(* Logix 5000 AddOnInstructionDefinition export AMCI_SMD23E2_Program_Assembed_Move; software revision 20.03 *)

ADD_ON_INSTRUCTION AMCI_SMD23E2_Program_Assembed_Move   (* revision 1.0, vendor AMCI *)
VAR_INPUT
   SMD23E2_Status_Word_0 : INT; {required}
        .8   // set when SMD23E2 is in Assembled Move mode
        .9   // set when the SMD23E2 is ready to receive an assembled move segment
   Number_of_Segments : DINT; {required}
   Segment_1_Distance : DINT; {required}
   Segment_1_Programmed_Speed : DINT; {required}
   Segment_1_Acceleration : INT; {required}
   Segment_1_Deceleration : INT; {required}
   Segment_2_Distance : DINT; {required}
   Segment_2_Programmed_Speed : DINT; {required}
   Segment_2_Acceleration : INT; {required}
   Segment_2_Deceleration : INT; {required}
   Segment_3_Distance : DINT; {required}
   Segment_3_Programmed_Speed : DINT; {required}
   Segment_3_Acceleration : INT; {required}
   Segment_3_Deceleration : INT; {required}
   Segment_4_Distance : DINT; {required}
   Segment_4_Programmed_Speed : DINT; {required}
   Segment_4_Acceleration : INT; {required}
   Segment_4_Deceleration : INT; {required}
   Segment_5_Distance : DINT; {required}
   Segment_5_Programmed_Speed : DINT; {required}
   Segment_5_Acceleration : INT; {required}
   Segment_5_Deceleration : INT; {required}
   Segment_6_Distance : DINT; {required}
   Segment_6_Programmed_Speed : DINT; {required}
   Segment_6_Acceleration : INT; {required}
   Segment_6_Deceleration : INT; {required}
   Segment_7_Distance : DINT; {required}
   Segment_7_Programmed_Speed : DINT; {required}
   Segment_7_Acceleration : INT; {required}
   Segment_7_Deceleration : INT; {required}
   Segment_8_Distance : DINT; {required}
   Segment_8_Programmed_Speed : DINT; {required}
   Segment_8_Acceleration : INT; {required}
   Segment_8_Deceleration : INT; {required}
   Segment_9_Distance : DINT; {required}
   Segment_9_Programmed_Speed : DINT; {required}
   Segment_9_Acceleration : INT; {required}
   Segment_9_Deceleration : INT; {required}
   Segment_10_Distance : DINT; {required}
   Segment_10_Programmed_Speed : DINT; {required}
   Segment_10_Acceleration : INT; {required}
   Segment_10_Deceleration : INT; {required}
   Segment_11_Distance : DINT; {required}
   Segment_11_Programmed_Speed : DINT; {required}
   Segment_11_Acceleration : INT; {required}
   Segment_11_Deceleration : INT; {required}
   Segment_12_Distance : DINT; {required}
   Segment_12_Programmed_Speed : DINT; {required}
   Segment_12_Acceleration : INT; {required}
   Segment_12_Deceleration : INT; {required}
   Segment_13_Distance : DINT; {required}
   Segment_13_Programmed_Speed : DINT; {required}
   Segment_13_Acceleration : INT; {required}
   Segment_13_Deceleration : INT; {required}
   Segment_14_Distance : DINT; {required}
   Segment_14_Programmed_Speed : DINT; {required}
   Segment_14_Acceleration : INT; {required}
   Segment_14_Deceleration : INT; {required}
   Segment_15_Distance : DINT; {required}
   Segment_15_Programmed_Speed : DINT; {required}
   Segment_15_Acceleration : INT; {required}
   Segment_15_Deceleration : INT; {required}
   Segment_16_Distance : DINT; {required}
   Segment_16_Programmed_Speed : DINT; {required}
   Segment_16_Acceleration : INT; {required}
   Segment_16_Deceleration : INT; {required}
END_VAR
VAR_IN_OUT
   AMCI_SMD23E2_output_data : _000A:SMD23E2_788832CB:O:0; {required}
END_VAR
VAR_OUTPUT
   Assembled_Move_Programmed : BOOL; {access Read Only, visible}
END_VAR
VAR
   command_data_block : INT[10];
        [0]   // Command Bits MSW
        [1]   // Command Bits LSW
        [2]   // Upper Target Position
        [3]   // Lower Target Position
        [4]   // Upper Programmed Speed
        [5]   // Lower Programmed Speed
   Assembled_Move_setup : INT[10] := ([0] := 2048, [1] := -32768); {access None}
   Assembled_Move_counter : COUNTER := (PRE := 5); {access None}
        .ACC   // Controls which segment is sent to the SMD23E2
   comment_coil : BOOL; {access None}
END_VAR

ROUTINE Logic   (* ladder *)
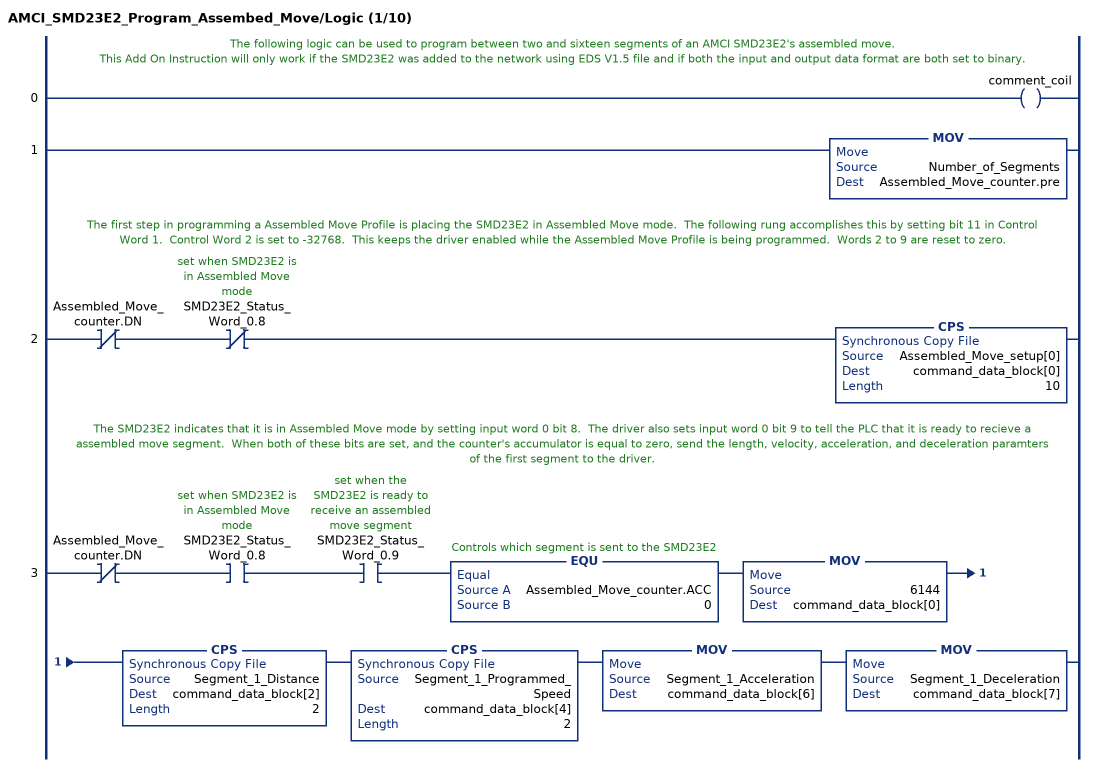
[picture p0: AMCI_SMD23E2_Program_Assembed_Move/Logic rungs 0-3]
   // The following logic can be used to program between two and sixteen segments of an AMCI SMD23E2's assembled move.
   // This Add On Instruction will only work if the SMD23E2 was added to the network using EDS V1.5 file and if both the input and output data format are both set to binary.
   0: OTE(comment_coil);
   1: MOV(Number_of_Segments,Assembled_Move_counter.pre);
   // The first step in programming a Assembled Move Profile is placing the SMD23E2 in Assembled Move mode.  The following rung accomplishes this by setting bit 11 in Control Word 1.  Control Word 2 is set to -32768.  This keeps the driver enabled while the Assembled Move Profile is being programmed.  Words 2 to 9 are reset to zero.
   2: XIO(Assembled_Move_counter.DN)XIO(SMD23E2_Status_Word_0.8)CPS(Assembled_Move_setup[0],command_data_block[0],10);
   // The SMD23E2 indicates that it is in Assembled Move mode by setting input word 0 bit 8.  The driver also sets input word 0 bit 9 to tell the PLC that it is ready to recieve a assembled move segment.  When both of these bits are set, and the counter's accumulator is equal to zero, send the length, velocity, acceleration, and deceleration paramters of the first segment to the driver.
   3: XIO(Assembled_Move_counter.DN)XIC(SMD23E2_Status_Word_0.8)XIC(SMD23E2_Status_Word_0.9)EQU(Assembled_Move_counter.ACC,0)MOV(6144,command_data_block[0])CPS(Segment_1_Distance,command_data_block[2],2)CPS(Segment_1_Programmed_Speed,command_data_block[4],2)MOV(Segment_1_Acceleration,command_data_block[6])MOV(Segment_1_Deceleration,command_data_block[7]);
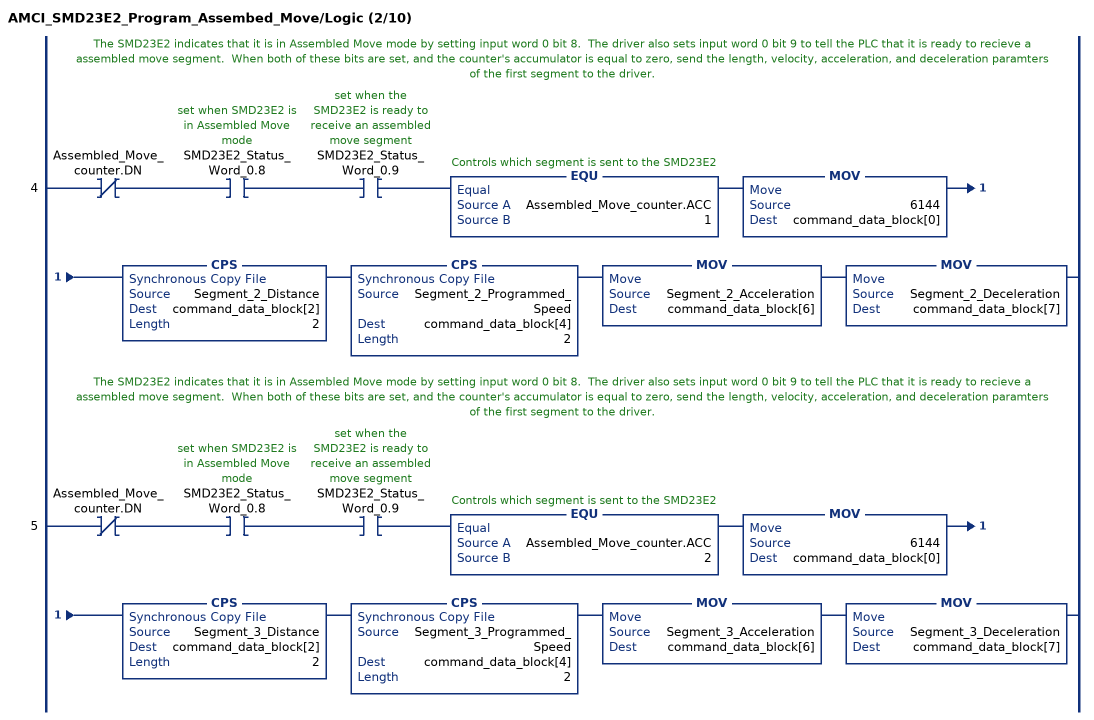
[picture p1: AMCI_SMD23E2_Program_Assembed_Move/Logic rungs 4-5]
   // The SMD23E2 indicates that it is in Assembled Move mode by setting input word 0 bit 8.  The driver also sets input word 0 bit 9 to tell the PLC that it is ready to recieve a assembled move segment.  When both of these bits are set, and the counter's accumulator is equal to zero, send the length, velocity, acceleration, and deceleration paramters of the first segment to the driver.
   4: XIO(Assembled_Move_counter.DN)XIC(SMD23E2_Status_Word_0.8)XIC(SMD23E2_Status_Word_0.9)EQU(Assembled_Move_counter.ACC,1)MOV(6144,command_data_block[0])CPS(Segment_2_Distance,command_data_block[2],2)CPS(Segment_2_Programmed_Speed,command_data_block[4],2)MOV(Segment_2_Acceleration,command_data_block[6])MOV(Segment_2_Deceleration,command_data_block[7]);
   // The SMD23E2 indicates that it is in Assembled Move mode by setting input word 0 bit 8.  The driver also sets input word 0 bit 9 to tell the PLC that it is ready to recieve a assembled move segment.  When both of these bits are set, and the counter's accumulator is equal to zero, send the length, velocity, acceleration, and deceleration paramters of the first segment to the driver.
   5: XIO(Assembled_Move_counter.DN)XIC(SMD23E2_Status_Word_0.8)XIC(SMD23E2_Status_Word_0.9)EQU(Assembled_Move_counter.ACC,2)MOV(6144,command_data_block[0])CPS(Segment_3_Distance,command_data_block[2],2)CPS(Segment_3_Programmed_Speed,command_data_block[4],2)MOV(Segment_3_Acceleration,command_data_block[6])MOV(Segment_3_Deceleration,command_data_block[7]);
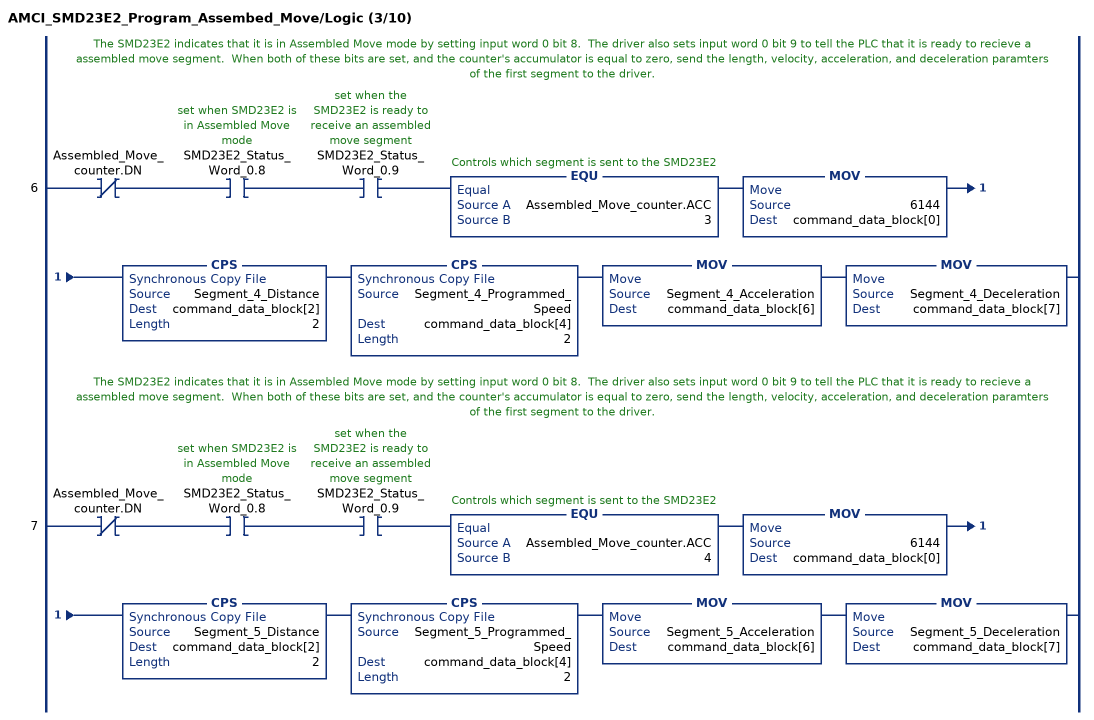
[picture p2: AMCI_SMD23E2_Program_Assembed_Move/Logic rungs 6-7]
   // The SMD23E2 indicates that it is in Assembled Move mode by setting input word 0 bit 8.  The driver also sets input word 0 bit 9 to tell the PLC that it is ready to recieve a assembled move segment.  When both of these bits are set, and the counter's accumulator is equal to zero, send the length, velocity, acceleration, and deceleration paramters of the first segment to the driver.
   6: XIO(Assembled_Move_counter.DN)XIC(SMD23E2_Status_Word_0.8)XIC(SMD23E2_Status_Word_0.9)EQU(Assembled_Move_counter.ACC,3)MOV(6144,command_data_block[0])CPS(Segment_4_Distance,command_data_block[2],2)CPS(Segment_4_Programmed_Speed,command_data_block[4],2)MOV(Segment_4_Acceleration,command_data_block[6])MOV(Segment_4_Deceleration,command_data_block[7]);
   // The SMD23E2 indicates that it is in Assembled Move mode by setting input word 0 bit 8.  The driver also sets input word 0 bit 9 to tell the PLC that it is ready to recieve a assembled move segment.  When both of these bits are set, and the counter's accumulator is equal to zero, send the length, velocity, acceleration, and deceleration paramters of the first segment to the driver.
   7: XIO(Assembled_Move_counter.DN)XIC(SMD23E2_Status_Word_0.8)XIC(SMD23E2_Status_Word_0.9)EQU(Assembled_Move_counter.ACC,4)MOV(6144,command_data_block[0])CPS(Segment_5_Distance,command_data_block[2],2)CPS(Segment_5_Programmed_Speed,command_data_block[4],2)MOV(Segment_5_Acceleration,command_data_block[6])MOV(Segment_5_Deceleration,command_data_block[7]);
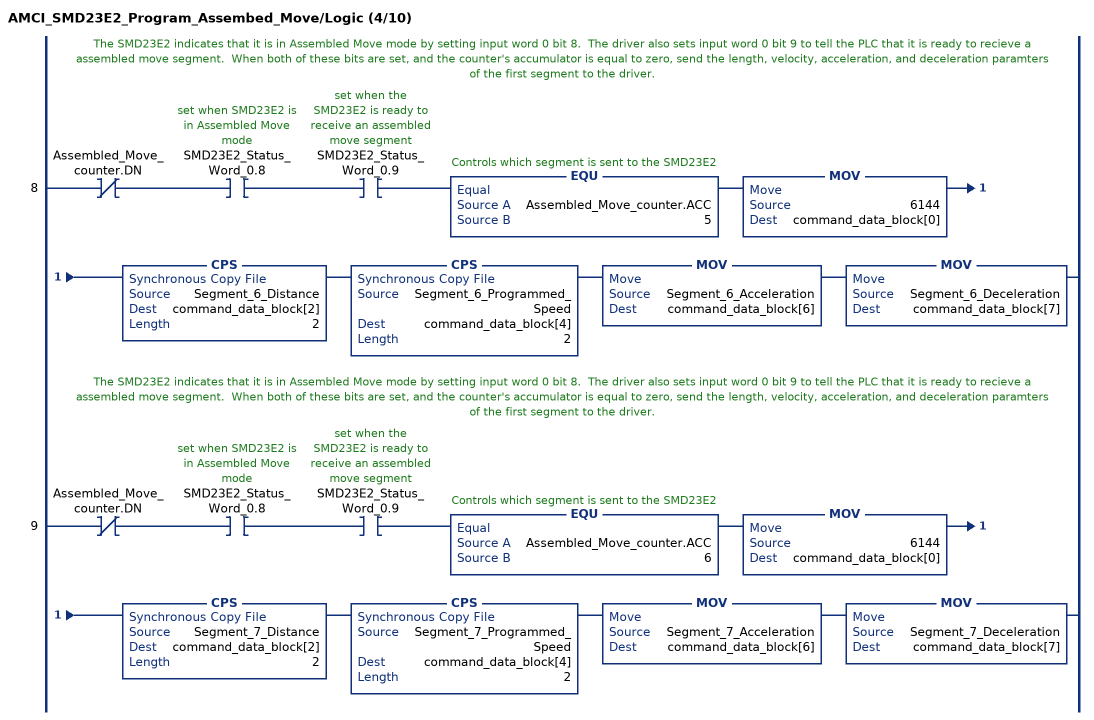
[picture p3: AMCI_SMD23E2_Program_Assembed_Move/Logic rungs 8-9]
   // The SMD23E2 indicates that it is in Assembled Move mode by setting input word 0 bit 8.  The driver also sets input word 0 bit 9 to tell the PLC that it is ready to recieve a assembled move segment.  When both of these bits are set, and the counter's accumulator is equal to zero, send the length, velocity, acceleration, and deceleration paramters of the first segment to the driver.
   8: XIO(Assembled_Move_counter.DN)XIC(SMD23E2_Status_Word_0.8)XIC(SMD23E2_Status_Word_0.9)EQU(Assembled_Move_counter.ACC,5)MOV(6144,command_data_block[0])CPS(Segment_6_Distance,command_data_block[2],2)CPS(Segment_6_Programmed_Speed,command_data_block[4],2)MOV(Segment_6_Acceleration,command_data_block[6])MOV(Segment_6_Deceleration,command_data_block[7]);
   // The SMD23E2 indicates that it is in Assembled Move mode by setting input word 0 bit 8.  The driver also sets input word 0 bit 9 to tell the PLC that it is ready to recieve a assembled move segment.  When both of these bits are set, and the counter's accumulator is equal to zero, send the length, velocity, acceleration, and deceleration paramters of the first segment to the driver.
   9: XIO(Assembled_Move_counter.DN)XIC(SMD23E2_Status_Word_0.8)XIC(SMD23E2_Status_Word_0.9)EQU(Assembled_Move_counter.ACC,6)MOV(6144,command_data_block[0])CPS(Segment_7_Distance,command_data_block[2],2)CPS(Segment_7_Programmed_Speed,command_data_block[4],2)MOV(Segment_7_Acceleration,command_data_block[6])MOV(Segment_7_Deceleration,command_data_block[7]);
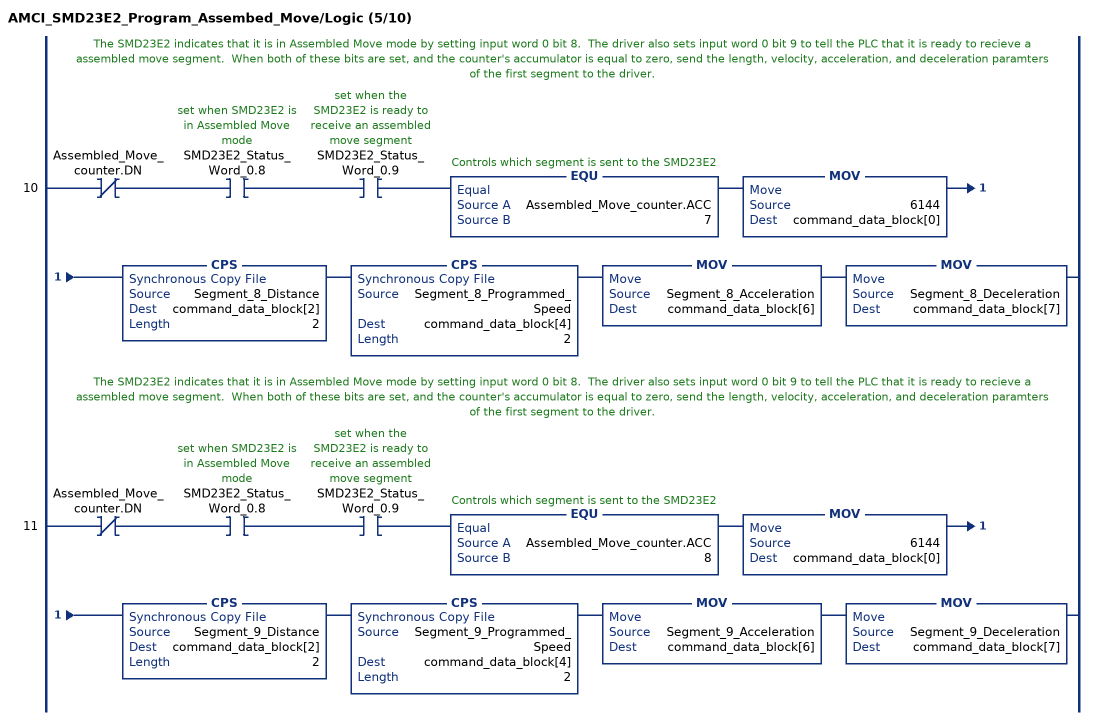
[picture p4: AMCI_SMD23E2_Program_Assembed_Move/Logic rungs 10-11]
   // The SMD23E2 indicates that it is in Assembled Move mode by setting input word 0 bit 8.  The driver also sets input word 0 bit 9 to tell the PLC that it is ready to recieve a assembled move segment.  When both of these bits are set, and the counter's accumulator is equal to zero, send the length, velocity, acceleration, and deceleration paramters of the first segment to the driver.
   10: XIO(Assembled_Move_counter.DN)XIC(SMD23E2_Status_Word_0.8)XIC(SMD23E2_Status_Word_0.9)EQU(Assembled_Move_counter.ACC,7)MOV(6144,command_data_block[0])CPS(Segment_8_Distance,command_data_block[2],2)CPS(Segment_8_Programmed_Speed,command_data_block[4],2)MOV(Segment_8_Acceleration,command_data_block[6])MOV(Segment_8_Deceleration,command_data_block[7]);
   // The SMD23E2 indicates that it is in Assembled Move mode by setting input word 0 bit 8.  The driver also sets input word 0 bit 9 to tell the PLC that it is ready to recieve a assembled move segment.  When both of these bits are set, and the counter's accumulator is equal to zero, send the length, velocity, acceleration, and deceleration paramters of the first segment to the driver.
   11: XIO(Assembled_Move_counter.DN)XIC(SMD23E2_Status_Word_0.8)XIC(SMD23E2_Status_Word_0.9)EQU(Assembled_Move_counter.ACC,8)MOV(6144,command_data_block[0])CPS(Segment_9_Distance,command_data_block[2],2)CPS(Segment_9_Programmed_Speed,command_data_block[4],2)MOV(Segment_9_Acceleration,command_data_block[6])MOV(Segment_9_Deceleration,command_data_block[7]);
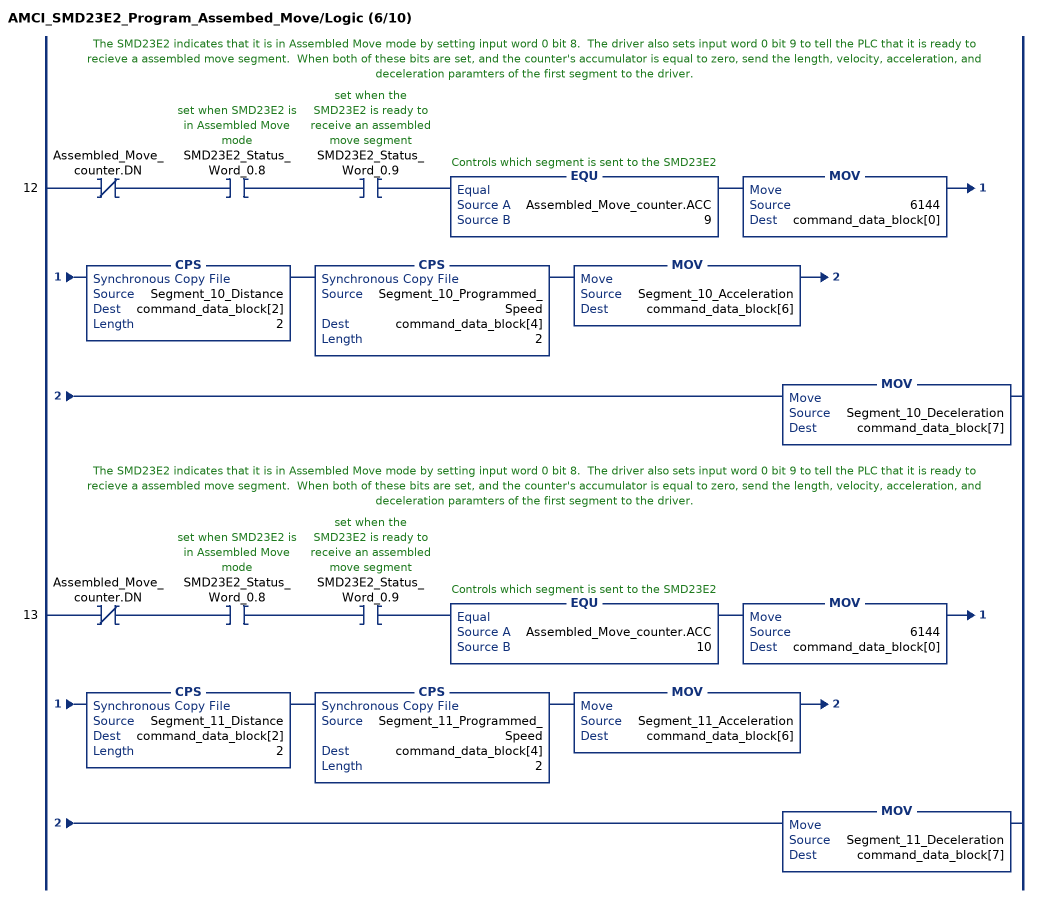
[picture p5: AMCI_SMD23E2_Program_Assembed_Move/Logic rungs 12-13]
   // The SMD23E2 indicates that it is in Assembled Move mode by setting input word 0 bit 8.  The driver also sets input word 0 bit 9 to tell the PLC that it is ready to recieve a assembled move segment.  When both of these bits are set, and the counter's accumulator is equal to zero, send the length, velocity, acceleration, and deceleration paramters of the first segment to the driver.
   12: XIO(Assembled_Move_counter.DN)XIC(SMD23E2_Status_Word_0.8)XIC(SMD23E2_Status_Word_0.9)EQU(Assembled_Move_counter.ACC,9)MOV(6144,command_data_block[0])CPS(Segment_10_Distance,command_data_block[2],2)CPS(Segment_10_Programmed_Speed,command_data_block[4],2)MOV(Segment_10_Acceleration,command_data_block[6])MOV(Segment_10_Deceleration,command_data_block[7]);
   // The SMD23E2 indicates that it is in Assembled Move mode by setting input word 0 bit 8.  The driver also sets input word 0 bit 9 to tell the PLC that it is ready to recieve a assembled move segment.  When both of these bits are set, and the counter's accumulator is equal to zero, send the length, velocity, acceleration, and deceleration paramters of the first segment to the driver.
   13: XIO(Assembled_Move_counter.DN)XIC(SMD23E2_Status_Word_0.8)XIC(SMD23E2_Status_Word_0.9)EQU(Assembled_Move_counter.ACC,10)MOV(6144,command_data_block[0])CPS(Segment_11_Distance,command_data_block[2],2)CPS(Segment_11_Programmed_Speed,command_data_block[4],2)MOV(Segment_11_Acceleration,command_data_block[6])MOV(Segment_11_Deceleration,command_data_block[7]);
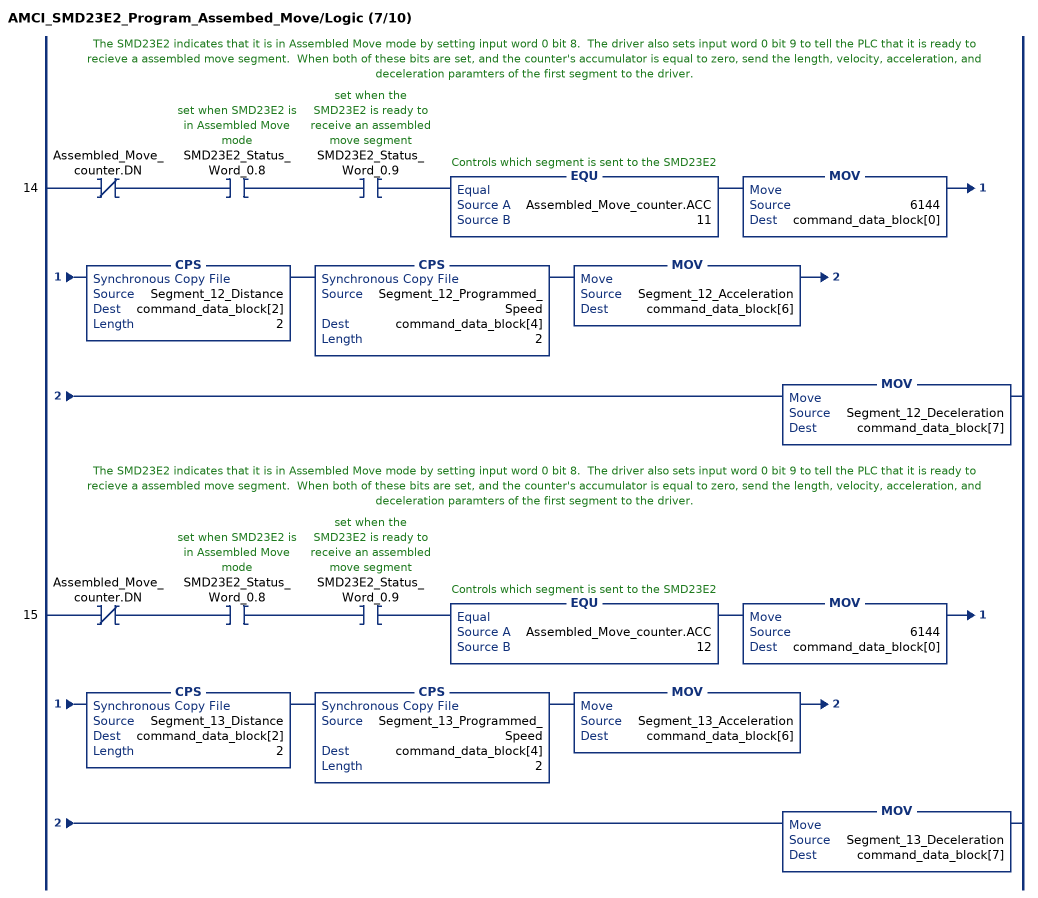
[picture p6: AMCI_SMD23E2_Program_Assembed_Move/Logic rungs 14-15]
   // The SMD23E2 indicates that it is in Assembled Move mode by setting input word 0 bit 8.  The driver also sets input word 0 bit 9 to tell the PLC that it is ready to recieve a assembled move segment.  When both of these bits are set, and the counter's accumulator is equal to zero, send the length, velocity, acceleration, and deceleration paramters of the first segment to the driver.
   14: XIO(Assembled_Move_counter.DN)XIC(SMD23E2_Status_Word_0.8)XIC(SMD23E2_Status_Word_0.9)EQU(Assembled_Move_counter.ACC,11)MOV(6144,command_data_block[0])CPS(Segment_12_Distance,command_data_block[2],2)CPS(Segment_12_Programmed_Speed,command_data_block[4],2)MOV(Segment_12_Acceleration,command_data_block[6])MOV(Segment_12_Deceleration,command_data_block[7]);
   // The SMD23E2 indicates that it is in Assembled Move mode by setting input word 0 bit 8.  The driver also sets input word 0 bit 9 to tell the PLC that it is ready to recieve a assembled move segment.  When both of these bits are set, and the counter's accumulator is equal to zero, send the length, velocity, acceleration, and deceleration paramters of the first segment to the driver.
   15: XIO(Assembled_Move_counter.DN)XIC(SMD23E2_Status_Word_0.8)XIC(SMD23E2_Status_Word_0.9)EQU(Assembled_Move_counter.ACC,12)MOV(6144,command_data_block[0])CPS(Segment_13_Distance,command_data_block[2],2)CPS(Segment_13_Programmed_Speed,command_data_block[4],2)MOV(Segment_13_Acceleration,command_data_block[6])MOV(Segment_13_Deceleration,command_data_block[7]);
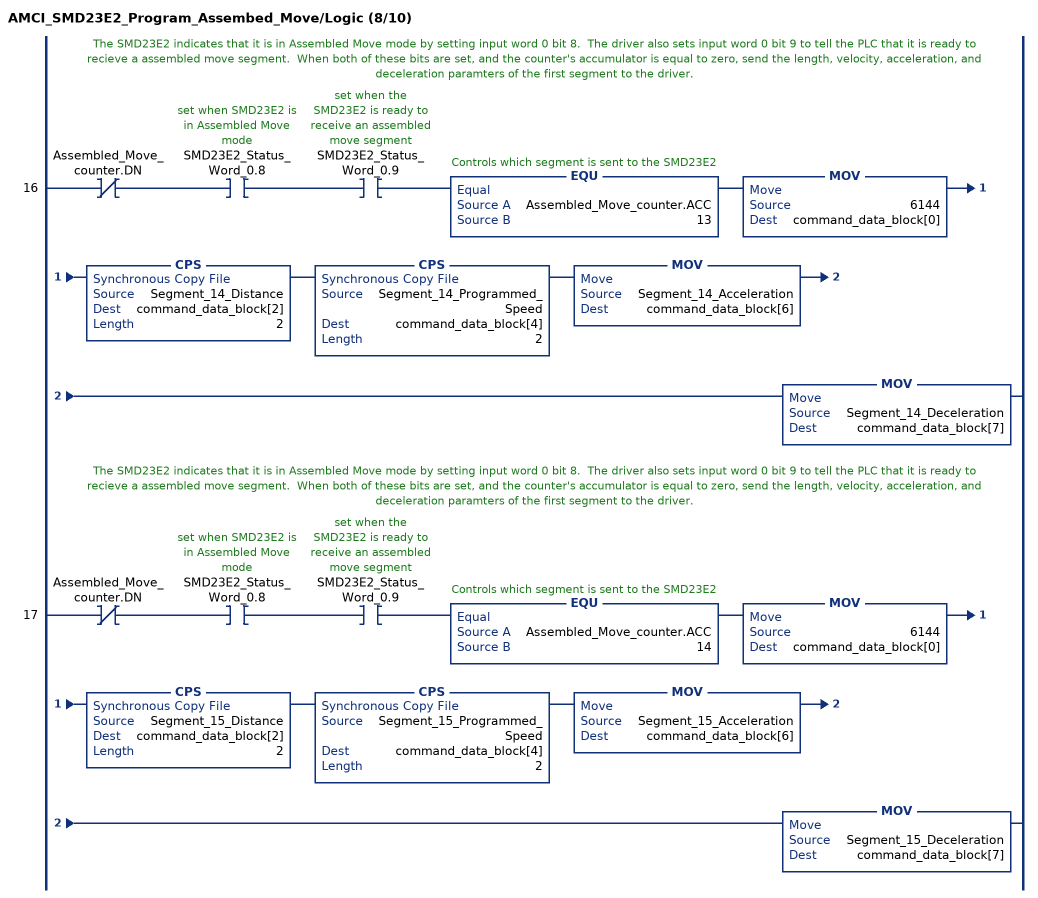
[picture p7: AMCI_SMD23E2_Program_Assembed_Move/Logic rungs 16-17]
   // The SMD23E2 indicates that it is in Assembled Move mode by setting input word 0 bit 8.  The driver also sets input word 0 bit 9 to tell the PLC that it is ready to recieve a assembled move segment.  When both of these bits are set, and the counter's accumulator is equal to zero, send the length, velocity, acceleration, and deceleration paramters of the first segment to the driver.
   16: XIO(Assembled_Move_counter.DN)XIC(SMD23E2_Status_Word_0.8)XIC(SMD23E2_Status_Word_0.9)EQU(Assembled_Move_counter.ACC,13)MOV(6144,command_data_block[0])CPS(Segment_14_Distance,command_data_block[2],2)CPS(Segment_14_Programmed_Speed,command_data_block[4],2)MOV(Segment_14_Acceleration,command_data_block[6])MOV(Segment_14_Deceleration,command_data_block[7]);
   // The SMD23E2 indicates that it is in Assembled Move mode by setting input word 0 bit 8.  The driver also sets input word 0 bit 9 to tell the PLC that it is ready to recieve a assembled move segment.  When both of these bits are set, and the counter's accumulator is equal to zero, send the length, velocity, acceleration, and deceleration paramters of the first segment to the driver.
   17: XIO(Assembled_Move_counter.DN)XIC(SMD23E2_Status_Word_0.8)XIC(SMD23E2_Status_Word_0.9)EQU(Assembled_Move_counter.ACC,14)MOV(6144,command_data_block[0])CPS(Segment_15_Distance,command_data_block[2],2)CPS(Segment_15_Programmed_Speed,command_data_block[4],2)MOV(Segment_15_Acceleration,command_data_block[6])MOV(Segment_15_Deceleration,command_data_block[7]);
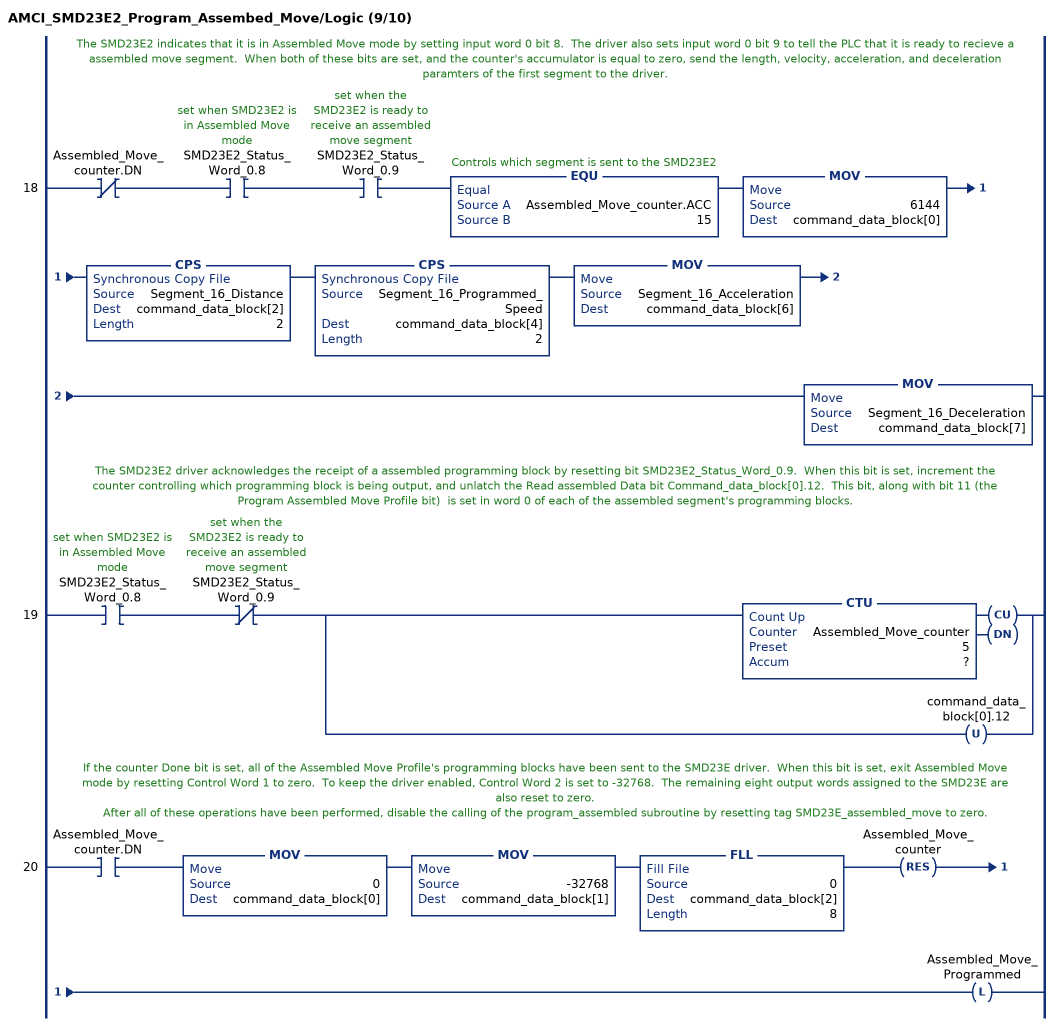
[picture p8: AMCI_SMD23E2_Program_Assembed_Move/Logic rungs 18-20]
   // The SMD23E2 indicates that it is in Assembled Move mode by setting input word 0 bit 8.  The driver also sets input word 0 bit 9 to tell the PLC that it is ready to recieve a assembled move segment.  When both of these bits are set, and the counter's accumulator is equal to zero, send the length, velocity, acceleration, and deceleration paramters of the first segment to the driver.
   18: XIO(Assembled_Move_counter.DN)XIC(SMD23E2_Status_Word_0.8)XIC(SMD23E2_Status_Word_0.9)EQU(Assembled_Move_counter.ACC,15)MOV(6144,command_data_block[0])CPS(Segment_16_Distance,command_data_block[2],2)CPS(Segment_16_Programmed_Speed,command_data_block[4],2)MOV(Segment_16_Acceleration,command_data_block[6])MOV(Segment_16_Deceleration,command_data_block[7]);
   // The SMD23E2 driver acknowledges the receipt of a assembled programming block by resetting bit SMD23E2_Status_Word_0.9.  When this bit is set, increment the counter controlling which programming block is being output, and unlatch the Read assembled Data bit Command_data_block[0].12.  This bit, along with bit 11 (the Program Assembled Move Profile bit)  is set in word 0 of each of the assembled segment's programming blocks.
   19: XIC(SMD23E2_Status_Word_0.8)XIO(SMD23E2_Status_Word_0.9)[CTU(Assembled_Move_counter,?,?) ,OTU(command_data_block[0].12) ];
   // If the counter Done bit is set, all of the Assembled Move Profile's programming blocks have been sent to the SMD23E driver.  When this bit is set, exit Assembled Move mode by resetting Control Word 1 to zero.  To keep the driver enabled, Control Word 2 is set to -32768.  The remaining eight output words assigned to the SMD23E are also reset to zero.
   // After all of these operations have been performed, disable the calling of the program_assembled subroutine by resetting tag SMD23E_assembled_move to zero.
   20: XIC(Assembled_Move_counter.DN)MOV(0,command_data_block[0])MOV(-32768,command_data_block[1])FLL(0,command_data_block[2],8)RES(Assembled_Move_counter)OTL(Assembled_Move_Programmed);
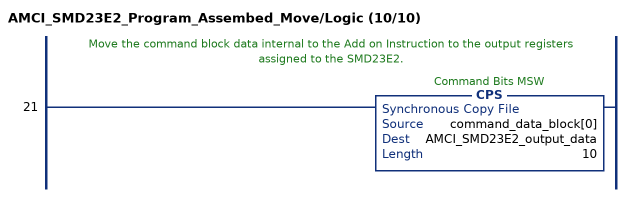
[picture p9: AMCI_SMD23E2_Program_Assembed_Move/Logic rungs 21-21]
   // Move the command block data internal to the Add on Instruction to the output registers assigned to the SMD23E2.
   21: CPS(command_data_block[0],AMCI_SMD23E2_output_data,10);
END_ROUTINE
END_ADD_ON_INSTRUCTION
